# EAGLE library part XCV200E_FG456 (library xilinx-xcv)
xcv200e_fg456 edit this description Auto generated by make-symbol-device-package-bsdl.ulp Rev. 26 Source: xcv200e_fg456.bsd
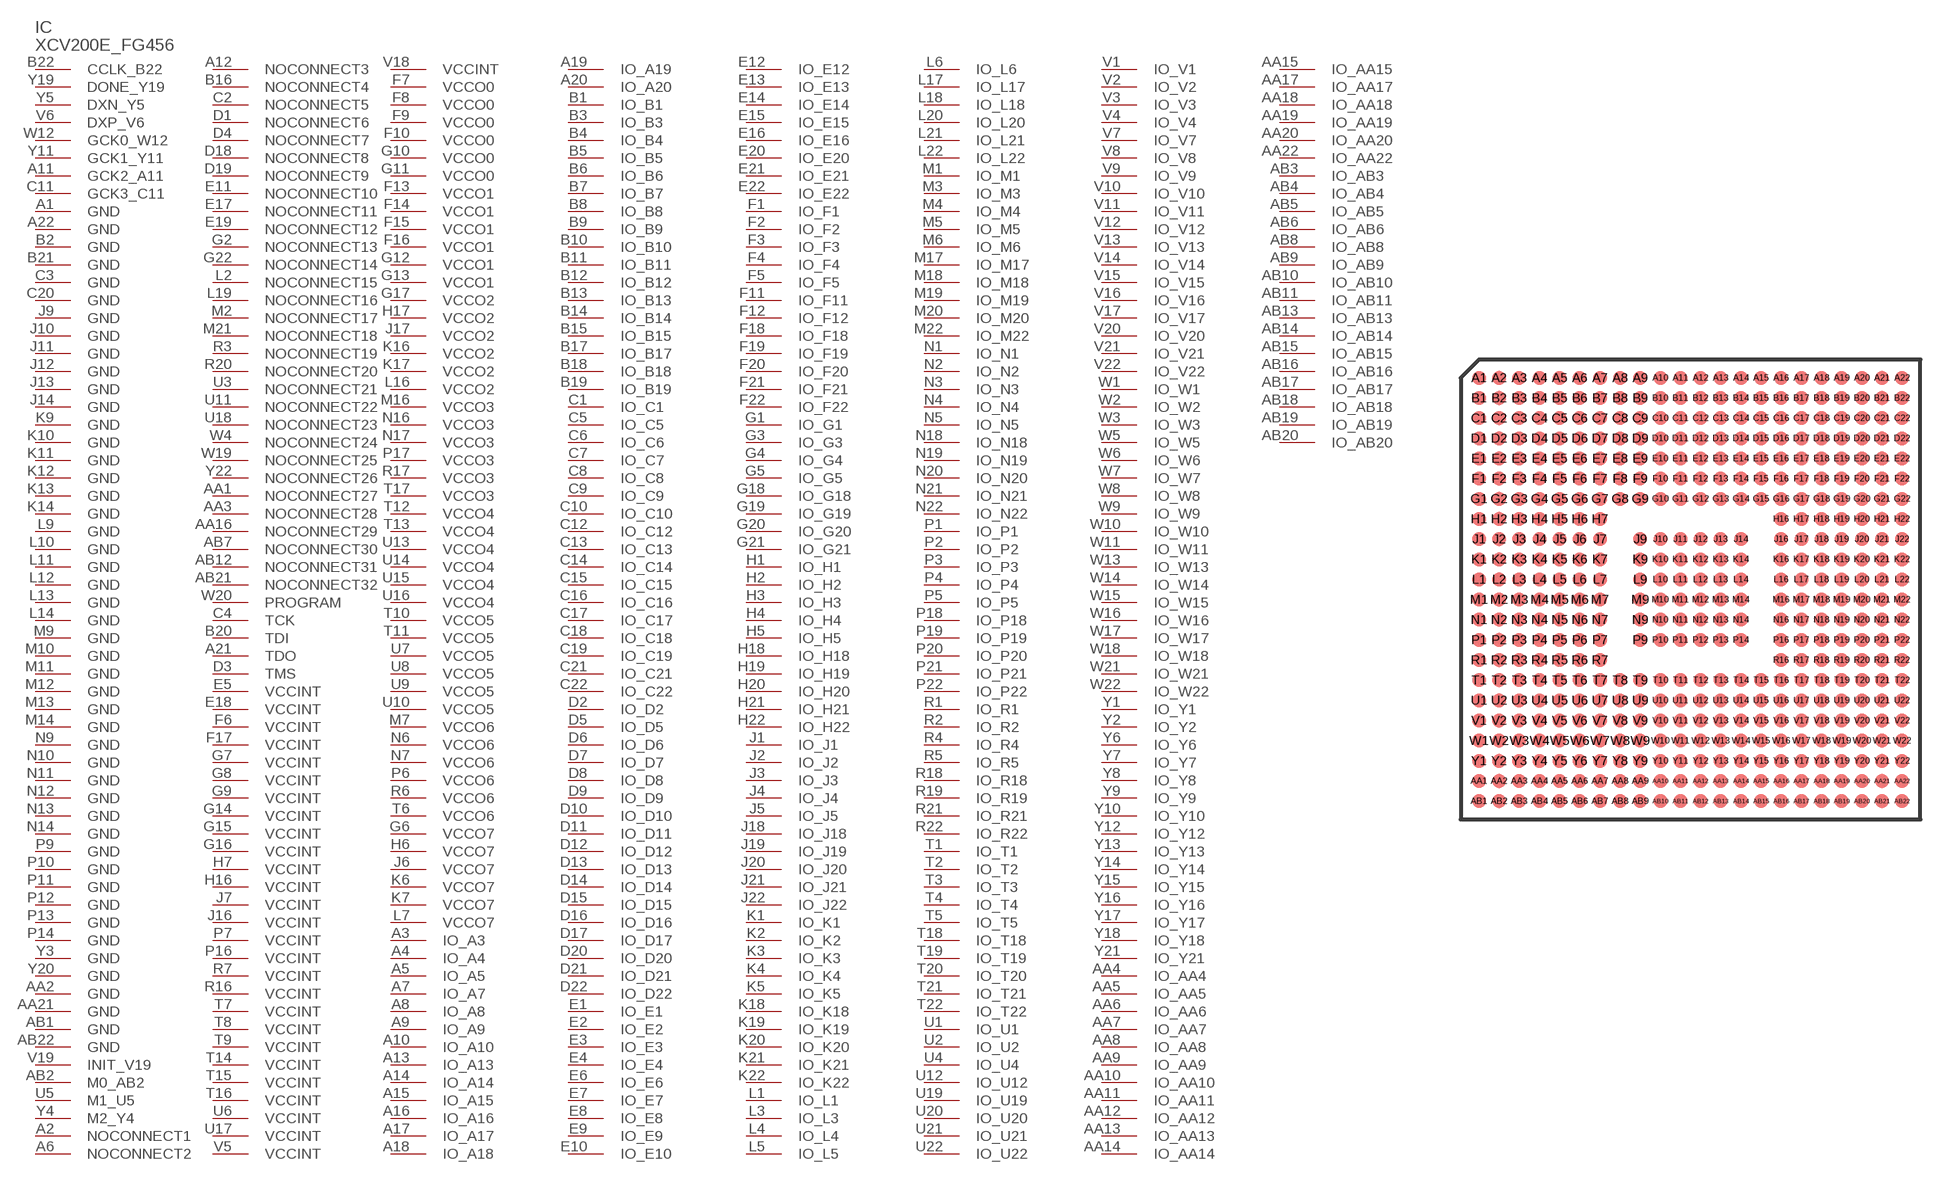
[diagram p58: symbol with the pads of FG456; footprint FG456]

Designator prefix IC

## XCV200E_FG456 (OC_FARNELL: unknown; OC_NEWARK: unknown)  [FG456]
A1  GND  pwr
A2  NOCONNECT1  pas
A3  IO_A3
A4  IO_A4
A5  IO_A5
A6  NOCONNECT2  pas
A7  IO_A7
A8  IO_A8
A9  IO_A9
A10  IO_A10
A11  GCK2_A11  in
A12  NOCONNECT3  pas
A13  IO_A13
A14  IO_A14
A15  IO_A15
A16  IO_A16
A17  IO_A17
A18  IO_A18
A19  IO_A19
A20  IO_A20
A21  TDO  out
A22  GND  pwr
AA1  NOCONNECT27  pas
AA2  GND  pwr
AA3  NOCONNECT28  pas
AA4  IO_AA4
AA5  IO_AA5
AA6  IO_AA6
AA7  IO_AA7
AA8  IO_AA8
AA9  IO_AA9
AA10  IO_AA10
AA11  IO_AA11
AA12  IO_AA12
AA13  IO_AA13
AA14  IO_AA14
AA15  IO_AA15
AA16  NOCONNECT29  pas
AA17  IO_AA17
AA18  IO_AA18
AA19  IO_AA19
AA20  IO_AA20
AA21  GND  pwr
AA22  IO_AA22
AB1  GND  pwr
AB2  M0_AB2  in
AB3  IO_AB3
AB4  IO_AB4
AB5  IO_AB5
AB6  IO_AB6
AB7  NOCONNECT30  pas
AB8  IO_AB8
AB9  IO_AB9
AB10  IO_AB10
AB11  IO_AB11
AB12  NOCONNECT31  pas
AB13  IO_AB13
AB14  IO_AB14
AB15  IO_AB15
AB16  IO_AB16
AB17  IO_AB17
AB18  IO_AB18
AB19  IO_AB19
AB20  IO_AB20
AB21  NOCONNECT32  pas
AB22  GND  pwr
B1  IO_B1
B2  GND  pwr
B3  IO_B3
B4  IO_B4
B5  IO_B5
B6  IO_B6
B7  IO_B7
B8  IO_B8
B9  IO_B9
B10  IO_B10
B11  IO_B11
B12  IO_B12
B13  IO_B13
B14  IO_B14
B15  IO_B15
B16  NOCONNECT4  pas
B17  IO_B17
B18  IO_B18
B19  IO_B19
B20  TDI  in
B21  GND  pwr
B22  CCLK_B22
C1  IO_C1
C2  NOCONNECT5  pas
C3  GND  pwr
C4  TCK  in
C5  IO_C5
C6  IO_C6
C7  IO_C7
C8  IO_C8
C9  IO_C9
C10  IO_C10
C11  GCK3_C11  in
C12  IO_C12
C13  IO_C13
C14  IO_C14
C15  IO_C15
C16  IO_C16
C17  IO_C17
C18  IO_C18
C19  IO_C19
C20  GND  pwr
C21  IO_C21
C22  IO_C22
D1  NOCONNECT6  pas
D2  IO_D2
D3  TMS  in
D4  NOCONNECT7  pas
D5  IO_D5
D6  IO_D6
D7  IO_D7
D8  IO_D8
D9  IO_D9
D10  IO_D10
D11  IO_D11
D12  IO_D12
D13  IO_D13
D14  IO_D14
D15  IO_D15
D16  IO_D16
D17  IO_D17
D18  NOCONNECT8  pas
D19  NOCONNECT9  pas
D20  IO_D20
D21  IO_D21
D22  IO_D22
E1  IO_E1
E2  IO_E2
E3  IO_E3
E4  IO_E4
E5  VCCINT  pwr
E6  IO_E6
E7  IO_E7
E8  IO_E8
E9  IO_E9
E10  IO_E10
E11  NOCONNECT10  pas
E12  IO_E12
E13  IO_E13
E14  IO_E14
E15  IO_E15
E16  IO_E16
E17  NOCONNECT11  pas
E18  VCCINT  pwr
E19  NOCONNECT12  pas
E20  IO_E20
E21  IO_E21
E22  IO_E22
F1  IO_F1
F2  IO_F2
F3  IO_F3
F4  IO_F4
F5  IO_F5
F6  VCCINT  pwr
F7  VCCO0  pwr
F8  VCCO0  pwr
F9  VCCO0  pwr
F10  VCCO0  pwr
F11  IO_F11
F12  IO_F12
F13  VCCO1  pwr
F14  VCCO1  pwr
F15  VCCO1  pwr
F16  VCCO1  pwr
F17  VCCINT  pwr
F18  IO_F18
F19  IO_F19
F20  IO_F20
F21  IO_F21
F22  IO_F22
G1  IO_G1
G2  NOCONNECT13  pas
G3  IO_G3
G4  IO_G4
G5  IO_G5
G6  VCCO7  pwr
G7  VCCINT  pwr
G8  VCCINT  pwr
G9  VCCINT  pwr
G10  VCCO0  pwr
G11  VCCO0  pwr
G12  VCCO1  pwr
G13  VCCO1  pwr
G14  VCCINT  pwr
G15  VCCINT  pwr
G16  VCCINT  pwr
G17  VCCO2  pwr
G18  IO_G18
G19  IO_G19
G20  IO_G20
G21  IO_G21
G22  NOCONNECT14  pas
H1  IO_H1
H2  IO_H2
H3  IO_H3
H4  IO_H4
H5  IO_H5
H6  VCCO7  pwr
H7  VCCINT  pwr
H16  VCCINT  pwr
H17  VCCO2  pwr
H18  IO_H18
H19  IO_H19
H20  IO_H20
H21  IO_H21
H22  IO_H22
J1  IO_J1
J2  IO_J2
J3  IO_J3
J4  IO_J4
J5  IO_J5
J6  VCCO7  pwr
J7  VCCINT  pwr
J9  GND  pwr
J10  GND  pwr
J11  GND  pwr
J12  GND  pwr
J13  GND  pwr
J14  GND  pwr
J16  VCCINT  pwr
J17  VCCO2  pwr
J18  IO_J18
J19  IO_J19
J20  IO_J20
J21  IO_J21
J22  IO_J22
K1  IO_K1
K2  IO_K2
K3  IO_K3
K4  IO_K4
K5  IO_K5
K6  VCCO7  pwr
K7  VCCO7  pwr
K9  GND  pwr
K10  GND  pwr
K11  GND  pwr
K12  GND  pwr
K13  GND  pwr
K14  GND  pwr
K16  VCCO2  pwr
K17  VCCO2  pwr
K18  IO_K18
K19  IO_K19
K20  IO_K20
K21  IO_K21
K22  IO_K22
L1  IO_L1
L2  NOCONNECT15  pas
L3  IO_L3
L4  IO_L4
L5  IO_L5
L6  IO_L6
L7  VCCO7  pwr
L9  GND  pwr
L10  GND  pwr
L11  GND  pwr
L12  GND  pwr
L13  GND  pwr
L14  GND  pwr
L16  VCCO2  pwr
L17  IO_L17
L18  IO_L18
L19  NOCONNECT16  pas
L20  IO_L20
L21  IO_L21
L22  IO_L22
M1  IO_M1
M2  NOCONNECT17  pas
M3  IO_M3
M4  IO_M4
M5  IO_M5
M6  IO_M6
M7  VCCO6  pwr
M9  GND  pwr
M10  GND  pwr
M11  GND  pwr
M12  GND  pwr
M13  GND  pwr
M14  GND  pwr
M16  VCCO3  pwr
M17  IO_M17
M18  IO_M18
M19  IO_M19
M20  IO_M20
M21  NOCONNECT18  pas
M22  IO_M22
N1  IO_N1
N2  IO_N2
N3  IO_N3
N4  IO_N4
N5  IO_N5
N6  VCCO6  pwr
N7  VCCO6  pwr
N9  GND  pwr
N10  GND  pwr
N11  GND  pwr
N12  GND  pwr
N13  GND  pwr
N14  GND  pwr
N16  VCCO3  pwr
N17  VCCO3  pwr
N18  IO_N18
N19  IO_N19
N20  IO_N20
N21  IO_N21
N22  IO_N22
P1  IO_P1
P2  IO_P2
P3  IO_P3
P4  IO_P4
P5  IO_P5
P6  VCCO6  pwr
P7  VCCINT  pwr
P9  GND  pwr
P10  GND  pwr
P11  GND  pwr
P12  GND  pwr
P13  GND  pwr
P14  GND  pwr
P16  VCCINT  pwr
P17  VCCO3  pwr
P18  IO_P18
P19  IO_P19
P20  IO_P20
P21  IO_P21
P22  IO_P22
R1  IO_R1
R2  IO_R2
R3  NOCONNECT19  pas
R4  IO_R4
R5  IO_R5
R6  VCCO6  pwr
R7  VCCINT  pwr
R16  VCCINT  pwr
R17  VCCO3  pwr
R18  IO_R18
R19  IO_R19
R20  NOCONNECT20  pas
R21  IO_R21
R22  IO_R22
T1  IO_T1
T2  IO_T2
T3  IO_T3
T4  IO_T4
T5  IO_T5
T6  VCCO6  pwr
T7  VCCINT  pwr
T8  VCCINT  pwr
T9  VCCINT  pwr
T10  VCCO5  pwr
T11  VCCO5  pwr
T12  VCCO4  pwr
T13  VCCO4  pwr
T14  VCCINT  pwr
T15  VCCINT  pwr
T16  VCCINT  pwr
T17  VCCO3  pwr
T18  IO_T18
T19  IO_T19
T20  IO_T20
T21  IO_T21
T22  IO_T22
U1  IO_U1
U2  IO_U2
U3  NOCONNECT21  pas
U4  IO_U4
U5  M1_U5  in
U6  VCCINT  pwr
U7  VCCO5  pwr
U8  VCCO5  pwr
U9  VCCO5  pwr
U10  VCCO5  pwr
U11  NOCONNECT22  pas
U12  IO_U12
U13  VCCO4  pwr
U14  VCCO4  pwr
U15  VCCO4  pwr
U16  VCCO4  pwr
U17  VCCINT  pwr
U18  NOCONNECT23  pas
U19  IO_U19
U20  IO_U20
U21  IO_U21
U22  IO_U22
V1  IO_V1
V2  IO_V2
V3  IO_V3
V4  IO_V4
V5  VCCINT  pwr
V6  DXP_V6  pas
V7  IO_V7
V8  IO_V8
V9  IO_V9
V10  IO_V10
V11  IO_V11
V12  IO_V12
V13  IO_V13
V14  IO_V14
V15  IO_V15
V16  IO_V16
V17  IO_V17
V18  VCCINT  pwr
V19  INIT_V19
V20  IO_V20
V21  IO_V21
V22  IO_V22
W1  IO_W1
W2  IO_W2
W3  IO_W3
W4  NOCONNECT24  pas
W5  IO_W5
W6  IO_W6
W7  IO_W7
W8  IO_W8
W9  IO_W9
W10  IO_W10
W11  IO_W11
W12  GCK0_W12  in
W13  IO_W13
W14  IO_W14
W15  IO_W15
W16  IO_W16
W17  IO_W17
W18  IO_W18
W19  NOCONNECT25  pas
W20  PROGRAM  in
W21  IO_W21
W22  IO_W22
Y1  IO_Y1
Y2  IO_Y2
Y3  GND  pwr
Y4  M2_Y4  in
Y5  DXN_Y5  pas
Y6  IO_Y6
Y7  IO_Y7
Y8  IO_Y8
Y9  IO_Y9
Y10  IO_Y10
Y11  GCK1_Y11  in
Y12  IO_Y12
Y13  IO_Y13
Y14  IO_Y14
Y15  IO_Y15
Y16  IO_Y16
Y17  IO_Y17
Y18  IO_Y18
Y19  DONE_Y19
Y20  GND  pwr
Y21  IO_Y21
Y22  NOCONNECT26  pas

## Footprint FG456 (pad centres in mm)
xcv150_fg456 edit this description Auto generated by make-symbol-device-package-bsdl.ulp Rev. 26 Source: xcv150_fg456.bsd
smd 0.7 x 0.7: A1 -10.5,10.5; A2 -9.5,10.5; A3 -8.5,10.5; A4 -7.5,10.5; A5 -6.5,10.5; A6 -5.5,10.5; A7 -4.5,10.5; A8 -3.5,10.5; A9 -2.5,10.5; A10 -1.5,10.5; A11 -0.5,10.5; A12 0.5,10.5; A13 1.5,10.5; A14 2.5,10.5; A15 3.5,10.5; A16 4.5,10.5; A17 5.5,10.5; A18 6.5,10.5; A19 7.5,10.5; A20 8.5,10.5; A21 9.5,10.5; A22 10.5,10.5; AA1 -10.5,-9.5; AA2 -9.5,-9.5; AA3 -8.5,-9.5; AA4 -7.5,-9.5; AA5 -6.5,-9.5; AA6 -5.5,-9.5; AA7 -4.5,-9.5; AA8 -3.5,-9.5; AA9 -2.5,-9.5; AA10 -1.5,-9.5; AA11 -0.5,-9.5; AA12 0.5,-9.5; AA13 1.5,-9.5; AA14 2.5,-9.5; AA15 3.5,-9.5; AA16 4.5,-9.5; AA17 5.5,-9.5; AA18 6.5,-9.5; AA19 7.5,-9.5; AA20 8.5,-9.5; AA21 9.5,-9.5; AA22 10.5,-9.5; AB1 -10.5,-10.5; AB2 -9.5,-10.5; AB3 -8.5,-10.5; AB4 -7.5,-10.5; AB5 -6.5,-10.5; AB6 -5.5,-10.5; AB7 -4.5,-10.5; AB8 -3.5,-10.5; AB9 -2.5,-10.5; AB10 -1.5,-10.5; AB11 -0.5,-10.5; AB12 0.5,-10.5; AB13 1.5,-10.5; AB14 2.5,-10.5; AB15 3.5,-10.5; AB16 4.5,-10.5; AB17 5.5,-10.5; AB18 6.5,-10.5; AB19 7.5,-10.5; AB20 8.5,-10.5; AB21 9.5,-10.5; AB22 10.5,-10.5; B1 -10.5,9.5; B2 -9.5,9.5; B3 -8.5,9.5; B4 -7.5,9.5; B5 -6.5,9.5; B6 -5.5,9.5; B7 -4.5,9.5; B8 -3.5,9.5; B9 -2.5,9.5; B10 -1.5,9.5; B11 -0.5,9.5; B12 0.5,9.5; B13 1.5,9.5; B14 2.5,9.5; B15 3.5,9.5; B16 4.5,9.5; B17 5.5,9.5; B18 6.5,9.5; B19 7.5,9.5; B20 8.5,9.5; B21 9.5,9.5; B22 10.5,9.5; C1 -10.5,8.5; C2 -9.5,8.5; C3 -8.5,8.5; C4 -7.5,8.5; C5 -6.5,8.5; C6 -5.5,8.5; C7 -4.5,8.5; C8 -3.5,8.5; C9 -2.5,8.5; C10 -1.5,8.5; C11 -0.5,8.5; C12 0.5,8.5; C13 1.5,8.5; C14 2.5,8.5; C15 3.5,8.5; C16 4.5,8.5; C17 5.5,8.5; C18 6.5,8.5; C19 7.5,8.5; C20 8.5,8.5; C21 9.5,8.5; C22 10.5,8.5; D1 -10.5,7.5; D2 -9.5,7.5; D3 -8.5,7.5; D4 -7.5,7.5; D5 -6.5,7.5; D6 -5.5,7.5; D7 -4.5,7.5; D8 -3.5,7.5; D9 -2.5,7.5; D10 -1.5,7.5; D11 -0.5,7.5; D12 0.5,7.5; D13 1.5,7.5; D14 2.5,7.5; D15 3.5,7.5; D16 4.5,7.5; D17 5.5,7.5; D18 6.5,7.5; D19 7.5,7.5; D20 8.5,7.5; D21 9.5,7.5; D22 10.5,7.5; E1 -10.5,6.5; E2 -9.5,6.5; E3 -8.5,6.5; E4 -7.5,6.5; E5 -6.5,6.5; E6 -5.5,6.5; E7 -4.5,6.5; E8 -3.5,6.5; E9 -2.5,6.5; E10 -1.5,6.5; E11 -0.5,6.5; E12 0.5,6.5; E13 1.5,6.5; E14 2.5,6.5; E15 3.5,6.5; E16 4.5,6.5; E17 5.5,6.5; E18 6.5,6.5; E19 7.5,6.5; E20 8.5,6.5; E21 9.5,6.5; E22 10.5,6.5; F1 -10.5,5.5; F2 -9.5,5.5; F3 -8.5,5.5; F4 -7.5,5.5; F5 -6.5,5.5; F6 -5.5,5.5; F7 -4.5,5.5; F8 -3.5,5.5; F9 -2.5,5.5; F10 -1.5,5.5; F11 -0.5,5.5; F12 0.5,5.5; F13 1.5,5.5; F14 2.5,5.5; F15 3.5,5.5; F16 4.5,5.5; F17 5.5,5.5; F18 6.5,5.5; F19 7.5,5.5; F20 8.5,5.5; F21 9.5,5.5; F22 10.5,5.5; G1 -10.5,4.5; G2 -9.5,4.5; G3 -8.5,4.5; G4 -7.5,4.5; G5 -6.5,4.5; G6 -5.5,4.5; G7 -4.5,4.5; G8 -3.5,4.5; G9 -2.5,4.5; G10 -1.5,4.5; G11 -0.5,4.5; G12 0.5,4.5; G13 1.5,4.5; G14 2.5,4.5; G15 3.5,4.5; G16 4.5,4.5; G17 5.5,4.5; G18 6.5,4.5; G19 7.5,4.5; G20 8.5,4.5; G21 9.5,4.5; G22 10.5,4.5; H1 -10.5,3.5; H2 -9.5,3.5; H3 -8.5,3.5; H4 -7.5,3.5; H5 -6.5,3.5; H6 -5.5,3.5; H7 -4.5,3.5; H16 4.5,3.5; H17 5.5,3.5; H18 6.5,3.5; H19 7.5,3.5; H20 8.5,3.5; H21 9.5,3.5; H22 10.5,3.5; J1 -10.5,2.5; J2 -9.5,2.5; J3 -8.5,2.5; J4 -7.5,2.5; J5 -6.5,2.5; J6 -5.5,2.5; J7 -4.5,2.5; J9 -2.5,2.5; J10 -1.5,2.5; J11 -0.5,2.5; J12 0.5,2.5; J13 1.5,2.5; J14 2.5,2.5; J16 4.5,2.5; J17 5.5,2.5; J18 6.5,2.5; J19 7.5,2.5; J20 8.5,2.5; J21 9.5,2.5; J22 10.5,2.5; K1 -10.5,1.5; K2 -9.5,1.5; K3 -8.5,1.5; K4 -7.5,1.5; K5 -6.5,1.5; K6 -5.5,1.5; K7 -4.5,1.5; K9 -2.5,1.5; K10 -1.5,1.5; K11 -0.5,1.5; K12 0.5,1.5; K13 1.5,1.5; K14 2.5,1.5; K16 4.5,1.5; K17 5.5,1.5; K18 6.5,1.5; K19 7.5,1.5; K20 8.5,1.5; K21 9.5,1.5; K22 10.5,1.5; L1 -10.5,0.5; L2 -9.5,0.5; L3 -8.5,0.5; L4 -7.5,0.5; L5 -6.5,0.5; L6 -5.5,0.5; L7 -4.5,0.5; L9 -2.5,0.5; L10 -1.5,0.5; L11 -0.5,0.5; L12 0.5,0.5; L13 1.5,0.5; L14 2.5,0.5; L16 4.5,0.5; L17 5.5,0.5; L18 6.5,0.5; L19 7.5,0.5; L20 8.5,0.5; L21 9.5,0.5; L22 10.5,0.5; M1 -10.5,-0.5; M2 -9.5,-0.5; M3 -8.5,-0.5; M4 -7.5,-0.5; M5 -6.5,-0.5; M6 -5.5,-0.5; M7 -4.5,-0.5; M9 -2.5,-0.5; M10 -1.5,-0.5; M11 -0.5,-0.5; M12 0.5,-0.5; M13 1.5,-0.5; M14 2.5,-0.5; M16 4.5,-0.5; M17 5.5,-0.5; M18 6.5,-0.5; M19 7.5,-0.5; M20 8.5,-0.5; M21 9.5,-0.5; M22 10.5,-0.5; N1 -10.5,-1.5; N2 -9.5,-1.5; N3 -8.5,-1.5; N4 -7.5,-1.5; N5 -6.5,-1.5; N6 -5.5,-1.5; N7 -4.5,-1.5; N9 -2.5,-1.5; N10 -1.5,-1.5; N11 -0.5,-1.5; N12 0.5,-1.5; N13 1.5,-1.5; N14 2.5,-1.5; N16 4.5,-1.5; N17 5.5,-1.5; N18 6.5,-1.5; N19 7.5,-1.5; N20 8.5,-1.5; N21 9.5,-1.5; N22 10.5,-1.5; P1 -10.5,-2.5; P2 -9.5,-2.5; P3 -8.5,-2.5; P4 -7.5,-2.5; P5 -6.5,-2.5; P6 -5.5,-2.5; P7 -4.5,-2.5; P9 -2.5,-2.5; P10 -1.5,-2.5; P11 -0.5,-2.5; P12 0.5,-2.5; P13 1.5,-2.5; P14 2.5,-2.5; P16 4.5,-2.5; P17 5.5,-2.5; P18 6.5,-2.5; P19 7.5,-2.5; P20 8.5,-2.5; P21 9.5,-2.5; P22 10.5,-2.5; R1 -10.5,-3.5; R2 -9.5,-3.5; R3 -8.5,-3.5; R4 -7.5,-3.5; R5 -6.5,-3.5; R6 -5.5,-3.5; R7 -4.5,-3.5; R16 4.5,-3.5; R17 5.5,-3.5; R18 6.5,-3.5; R19 7.5,-3.5; R20 8.5,-3.5; R21 9.5,-3.5; R22 10.5,-3.5; T1 -10.5,-4.5; T2 -9.5,-4.5; T3 -8.5,-4.5; T4 -7.5,-4.5; T5 -6.5,-4.5; T6 -5.5,-4.5; T7 -4.5,-4.5; T8 -3.5,-4.5; T9 -2.5,-4.5; T10 -1.5,-4.5; T11 -0.5,-4.5; T12 0.5,-4.5; T13 1.5,-4.5; T14 2.5,-4.5; T15 3.5,-4.5; T16 4.5,-4.5; T17 5.5,-4.5; T18 6.5,-4.5; T19 7.5,-4.5; T20 8.5,-4.5; T21 9.5,-4.5; T22 10.5,-4.5; U1 -10.5,-5.5; U2 -9.5,-5.5; U3 -8.5,-5.5; U4 -7.5,-5.5; U5 -6.5,-5.5; U6 -5.5,-5.5; U7 -4.5,-5.5; U8 -3.5,-5.5; U9 -2.5,-5.5; U10 -1.5,-5.5; U11 -0.5,-5.5; U12 0.5,-5.5; U13 1.5,-5.5; U14 2.5,-5.5; U15 3.5,-5.5; U16 4.5,-5.5; U17 5.5,-5.5; U18 6.5,-5.5; U19 7.5,-5.5; U20 8.5,-5.5; U21 9.5,-5.5; U22 10.5,-5.5; V1 -10.5,-6.5; V2 -9.5,-6.5; V3 -8.5,-6.5; V4 -7.5,-6.5; V5 -6.5,-6.5; V6 -5.5,-6.5; V7 -4.5,-6.5; V8 -3.5,-6.5; V9 -2.5,-6.5; V10 -1.5,-6.5; V11 -0.5,-6.5; V12 0.5,-6.5; V13 1.5,-6.5; V14 2.5,-6.5; V15 3.5,-6.5; V16 4.5,-6.5; V17 5.5,-6.5; V18 6.5,-6.5; V19 7.5,-6.5; V20 8.5,-6.5; V21 9.5,-6.5; V22 10.5,-6.5; W1 -10.5,-7.5; W2 -9.5,-7.5; W3 -8.5,-7.5; W4 -7.5,-7.5; W5 -6.5,-7.5; W6 -5.5,-7.5; W7 -4.5,-7.5; W8 -3.5,-7.5; W9 -2.5,-7.5; W10 -1.5,-7.5; W11 -0.5,-7.5; W12 0.5,-7.5; W13 1.5,-7.5; W14 2.5,-7.5; W15 3.5,-7.5; W16 4.5,-7.5; W17 5.5,-7.5; W18 6.5,-7.5; W19 7.5,-7.5; W20 8.5,-7.5; W21 9.5,-7.5; W22 10.5,-7.5; Y1 -10.5,-8.5; Y2 -9.5,-8.5; Y3 -8.5,-8.5; Y4 -7.5,-8.5; Y5 -6.5,-8.5; Y6 -5.5,-8.5; Y7 -4.5,-8.5; Y8 -3.5,-8.5; Y9 -2.5,-8.5; Y10 -1.5,-8.5; Y11 -0.5,-8.5; Y12 0.5,-8.5; Y13 1.5,-8.5; Y14 2.5,-8.5; Y15 3.5,-8.5; Y16 4.5,-8.5; Y17 5.5,-8.5; Y18 6.5,-8.5; Y19 7.5,-8.5; Y20 8.5,-8.5; Y21 9.5,-8.5; Y22 10.5,-8.5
